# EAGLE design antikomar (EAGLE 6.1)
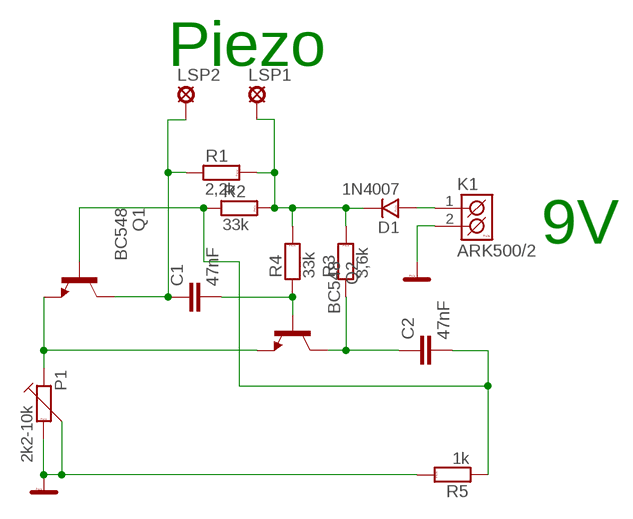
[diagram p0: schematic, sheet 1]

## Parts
C1  47nF  KERAMICKYRM5  [KERAMICKY_RM5]
C2  47nF  KERAMICKYRM5  [KERAMICKY_RM5]
D1  1N4007  1N4007_10  [DO41]
K1  ARK500/2  [ARK500/2]
LSP1  SE14  [SE14]
LSP2  SE14  [SE14]
P1  2k2-10k  TRIMRPT10V  [PT10V]
Q1  BC548  [TO92-EBC]
Q2  BC548  [TO92-EBC]
R1  2,2k  2K2  [R_7,5]
R2  33k  33K  [R_7,5]
R3  3,6k  33K  [R_7,5]
R4  33k  33K  [R_7,5]
R5  1k  33K  [R_7,5]

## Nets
GND: K1.2(K2) P1.2 P1.3 R5.2
N$1: C2.P$2 Q1.B R2.1 R5.1
N$2: C2.P$1 Q2.C R3.1
N$3: D1.A K1.1(K1)
N$5: C1.P$1 LSP2.MP Q1.C R1.1
N$6: D1.K LSP1.MP R1.2 R2.2 R3.2 R4.2
N$7: P1.1 Q1.E Q2.E
N$8: C1.P$2 Q2.B R4.1

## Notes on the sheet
- Piezo
- 9V

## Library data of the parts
C1 C2 = #Kondenzatory:KERAMICKY
D1 = #PaJa_30:1N4007: Usmernovaci dioda - 1A, 1000V
K1 = #PaJa_konektory:ARK500/2: Svorkovnice - roztec 5mm - dvojita
LSP1 LSP2 = solpad:SE14: SOLDER PAD
P1 = #PaJa_30:TRIMR: Trimr
Q1 Q2 = transistor-npn:BC548*: NPN Transistor
R1 = #PaJa_R:2K2
R2-R5 = #PaJa_R:33K

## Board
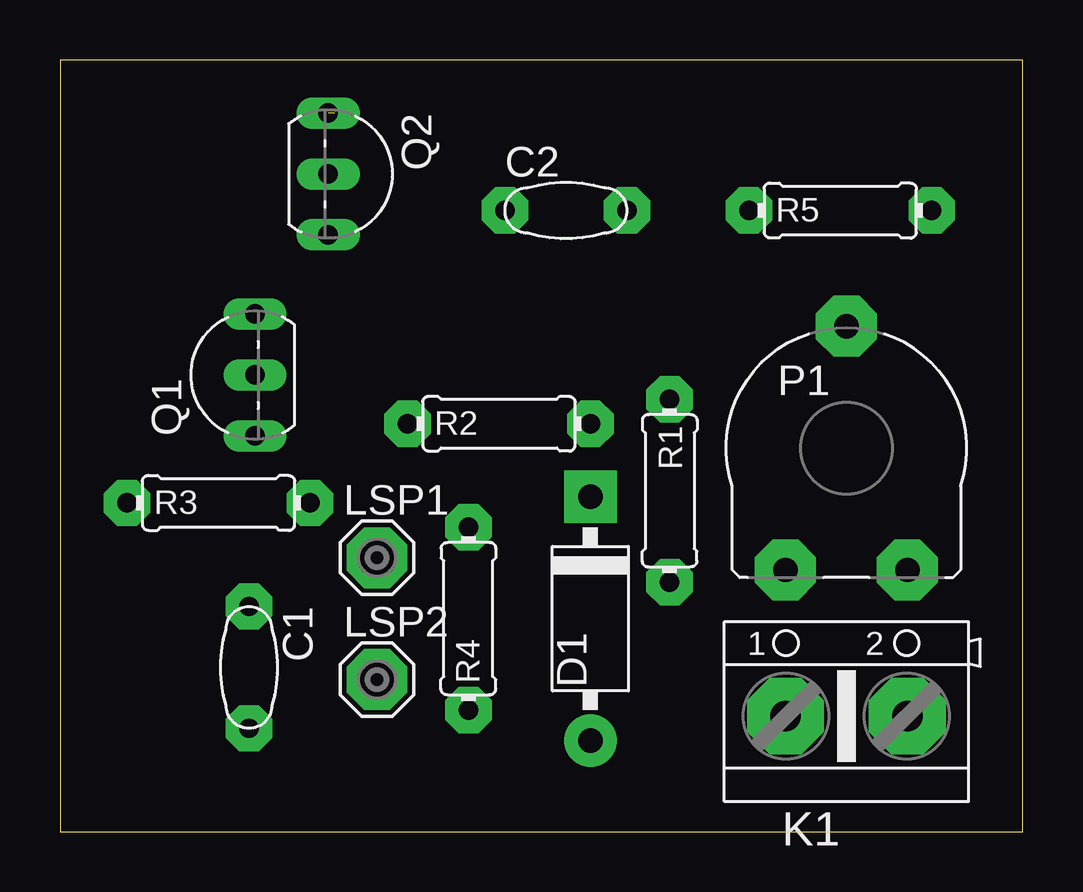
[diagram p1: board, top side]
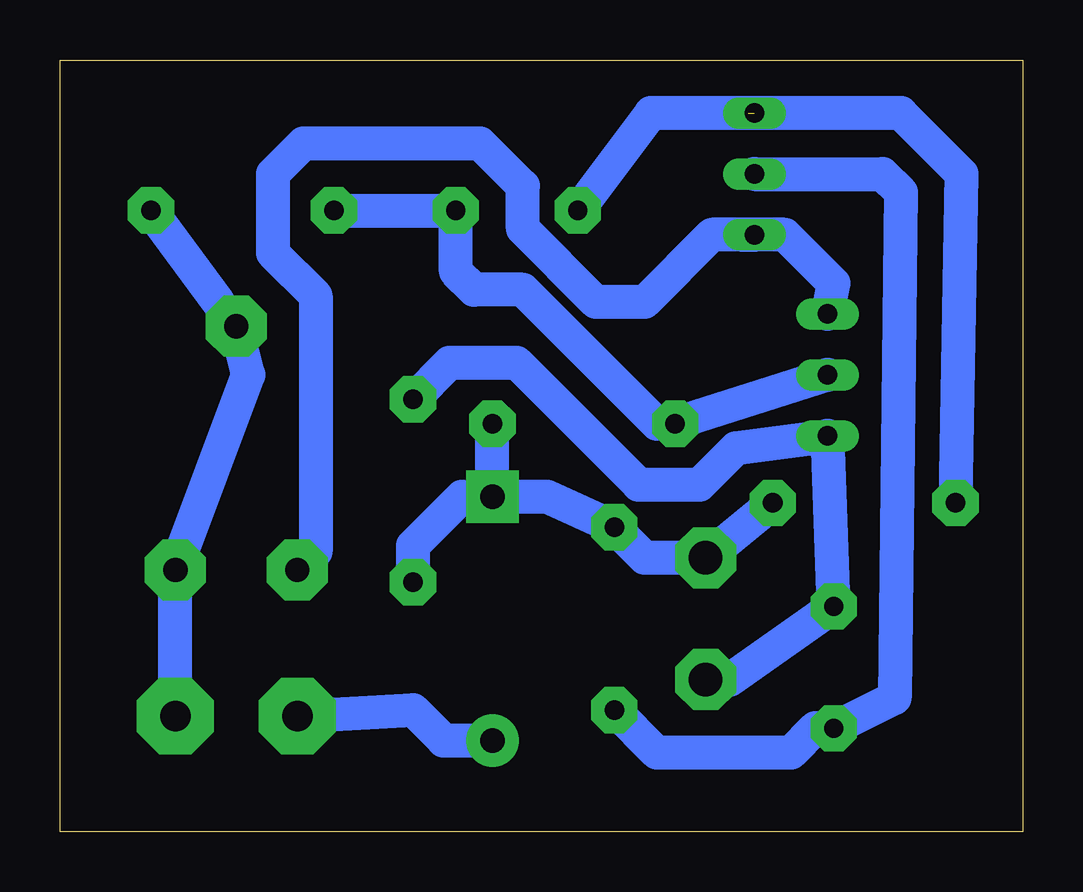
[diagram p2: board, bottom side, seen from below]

Size 40.11 x 32.18 mm. Coordinates in mm from the lower left corner, seen from the top.
Outline: 0,0 40.11,0 40.11,32.18 0,32.18 0,0
Copper layers (1*16): Top 0.035mm / dielectric 1.5mm / Bottom 0.035mm
Design rules: minimum track width 10mil, minimum drill 24mil, track to track 8mil, track to pad 8mil, pad to pad 8mil, via to via 8mil, smd to smd 8mil, copper to edge 40mil, drill to drill 8mil, minimum pad ring 10mil, minimum via ring 8mil, stop-mask expansion 4mil, vias tented up to drill 0mil, thermal gap 10mil

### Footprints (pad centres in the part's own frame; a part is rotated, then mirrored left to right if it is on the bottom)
KERAMICKY_RM5 = drill 0.8 pad 1.93 octagon: P$1 -2.54,0; P$2 2.54,0
DO41 = drill 1.016 pad 2.184: A -5.08,0 | drill 1.016 pad 2.184 square: K 5.08,0
ARK500/2 = drill 1.27 pad 3.2 octagon: 1 -2.54,0; 2 2.54,0
SE14 = drill 1.397 pad 2.54 octagon: MP 0,0
PT10V = drill 1.016 pad 2.54 octagon: 1 -2.54,-5.08; 2 2.54,-5.08; 3 0,5.08
TO92-EBC = drill 0.813 long: B 0,-1.27; C -2.54,-1.27; E 2.54,-1.27
R_7,5 = drill 0.813 pad 1.93 octagon: 1 -3.81,0; 2 3.81,0

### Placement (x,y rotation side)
C1  7.87,6.86 270 top
C2  21.08,25.91 0 top
D1  22.1,8.89 90 top
K1  32.77,4.83 0 top
LSP1  13.21,11.43 0 top
LSP2  13.21,6.35 0 top
P1  32.77,16 0 top
Q1  6.86,19.05 90 top
Q2  12.45,27.43 270 top
R1  25.4,14.22 270 top
R2  18.29,17.02 0 top
R3  6.6,13.72 0 top
R4  17.02,8.89 90 top
R5  32.51,25.91 0 top

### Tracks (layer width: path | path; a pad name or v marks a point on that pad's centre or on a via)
GND
  Bottom 1.422: K1.2 P1.2 32.26,19.05 P1.3 33.53,22.1 R5.2
N$1
  Bottom 1.422: Q1.B R2.1 15.24,17.02 20.83,22.61 22.86,22.61 23.62,23.37 C2.P$2 R5.1
N$2  (1 unrouted)
  Bottom 1.422: R3.1 2.54,27.43 5.08,29.97 Q2.C | Q2.C 11.43,29.97 | Q2.C 15.49,29.97 C2.P$1
N$3
  Bottom 1.422: K1.1 25.4,5.08 24.13,3.81 D1.A
N$5
  Bottom 1.422: LSP2.MP 12.19,6.35 C1.P$1 Q1.C 11.94,16 13.46,14.48 16,14.48 21.08,19.56 23.88,19.56 R1.1
N$6
  Bottom 1.422: R3.2 LSP1.MP 15.75,11.43 R4.2 19.81,13.97 D1.K 22.1,14.22 | R1.2 25.4,11.94 23.37,13.97 22.35,13.97 22.1,14.22 | 22.1,14.22 R2.2
N$7
  Bottom 1.422: Q1.E 7.87,22.86 9.91,24.89 Q2.E | 11.68,24.89 Q2.E | Q2.E 12.95,24.89 15.75,22.1 17.78,22.1 20.83,25.15 20.83,26.92 22.61,28.7 29.97,28.7 31.24,27.43 31.24,24.13 29.46,22.35 29.46,11.68 P1.1
N$8
  Bottom 1.422: Q2.B 5.84,27.43 5.08,26.67 5.33,5.59 C1.P$2 8.64,4.32 9.65,3.3 15.24,3.3 R4.1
